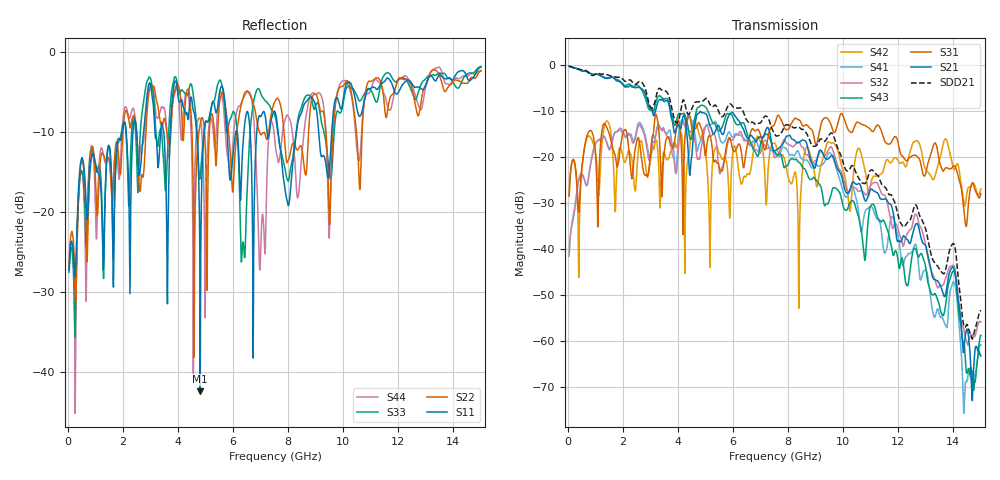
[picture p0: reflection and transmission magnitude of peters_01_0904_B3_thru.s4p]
# MHZ S RI R 50.00
! FREQ  S11  S12  S13  S14
!  S21  S22  S23  S24
!  S31  S32  S33  S34
!  S41  S42  S43  S44
!  REAL  IMAG  REAL  IMAG  REAL  IMAG  REAL  IMAG
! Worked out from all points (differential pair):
!   1496 points, 50 MHz to 15 GHz, reference 50 ohm
!   strongest paths, dB at 50 MHz, 3.79 GHz, 7.53 GHz, 11.27 GHz, 15 GHz:
!     S21: -0.2, -12.1, -18.6, -28.0, -63.3
!     S31: -28.5, -17.5, -12.5, -13.1, -27.9
!     S43: -0.2, -11.2, -18.9, -33.4, -58.8
!     S32: -41.5, -19.3, -20.1, -26.0, -55.9
!     S41: -41.4, -17.3, -19.2, -33.7, -61.0
!     S42: -28.5, -18.5, -17.1, -24.1, -26.9
!   taken as a pair (ports 1,3 in; 2,4 out), SDD21 dB: -0.2, -9.7, -15.2, -24.1, -53.5
!   lowest |S11| = -42.4 dB at 4.81 GHz (marker M1), VSWR 1.02, Z = 50.8 + j0.0143 ohm
!   |S11| at or under -10 dB: start of sweep to 1.973 GHz; 7.637 GHz to 8.302 GHz (664.6 MHz wide, 8.34 % of centre); 9.113 GHz to 9.584 GHz (471.1 MHz wide, 5.04 % of centre)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
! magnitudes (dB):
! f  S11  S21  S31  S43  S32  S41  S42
! 50 MHz  -27.2  -0.2  -28.5  -0.2  -41.5  -41.4  -28.5
! 1.08 GHz  -14.9  -2.0  -32.9  -2.0  -16.4  -16.5  -23.5
! 2.97 GHz  -3.8  -9.2  -21.4  -9.8  -20.8  -19.9  -22.1
! 4.81 GHz  -42.4  -10.1  -13.1  -8.8  -19.8  -16.7  -16.0
! 8.4 GHz  -8.2  -16.8  -11.9  -21.1  -16.8  -19.2  -42.4
! 9.56 GHz  -11.3  -19.7  -13.0  -28.2  -17.8  -19.3  -17.0
! 15 GHz  -1.9  -63.3  -27.9  -58.8  -55.9  -61.0  -26.9
